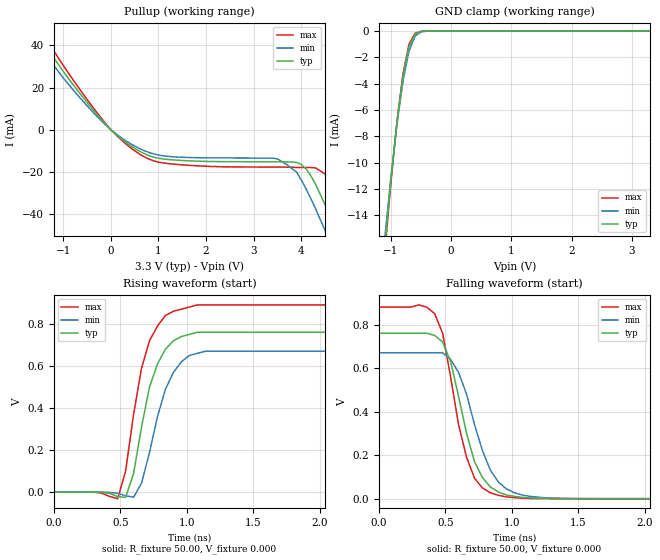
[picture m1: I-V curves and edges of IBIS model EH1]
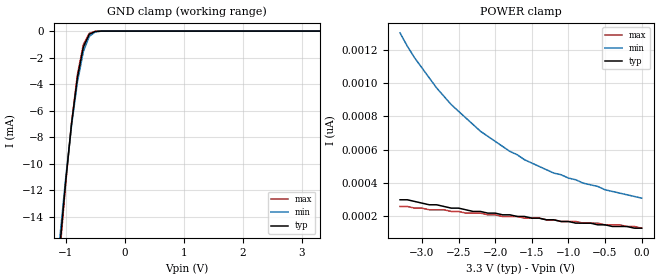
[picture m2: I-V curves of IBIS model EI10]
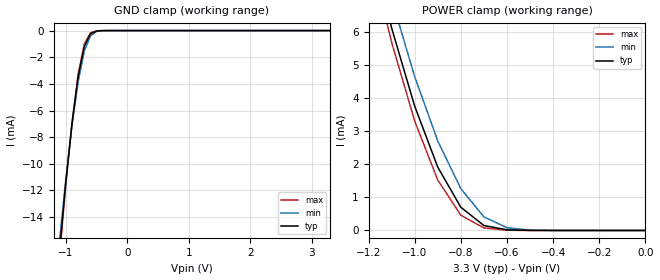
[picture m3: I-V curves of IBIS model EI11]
|   * fg1904b1.ibs * IBIS 2.1 Model file
| Rev History
| Rev No.   Description
| 1.0   3/22/07   Initial release with Updated Parasitic Parameters
|   Derived from fg1904ak ibis file
[IBIS Ver]   2.1
[Comment char]  |_char
[File name]   fg1904b1.ibs
[Date]   March 22, 2007
[File Rev]   1.0
[Source]   Originated at Integrated Device Technology, Inc.
[Disclaimer] (C) Copyright Integrated Device Technology, Inc. 2007
   All rights reserved
 hereby grants the user of this IBIS model a non-exclusive,
nontransferable license to use this IBIS model under the following terms.
Before using this IBIS model, the user should read this license.
If the user does not accept these terms,  the IBIS model should be
returned to IDT within 30 days.
   The user is granted this license only to use the IBIS model and
is not granted rights to sell, load, rent, lease or license the IBIS
model in whole or in part, or in modified form to anyone other than
user. User may modify the IBIS model to suit its specific
applications but rights to derivative works and such modifications
shall belong to IDT.
   This IBIS model is provided on an "AS IS" basis and IDT makes
absolutely no warranty with respect to the information contained
herein. IDT DISCLAIMS AND CUSTOMER WAIVES ALL WARRANTIES, EXPRESS
OR IMPLIED, INCLUDING WARRANTIES OF MERCHANTABILITY OR FITNESS FOR
A PARTICULAR PURPOSE. The entire risk as to quality and performance
is with the Customer. ACCORDINGLY, IN NO EVENT SHALL THE COMPANY BE
LIABLE FOR ANY DAMAGES, WHETHER IN CONTRACT OR TORT,INCLUDING ANY
LOST PROFITS OR OTHER INCIDENTAL, CONSEQUENTIAL, EXEMPLARY, OR
PUNITIVE DAMAGES ARISING OUT OF THE USE OR APPLICATION OF THE IBIS
model provided in this package. Further, IDT reserves the right to
make changes without notice to any product herein to improve
reliability, function, or design. IDT does not convey any license
under patent rights or any other intellectual property rights,
including those of third parties.
   IDT is not obligated to provide maintenance or support
for the licensed IBIS model.
|   COMPONENT: ICS9FG1904
[Component]   ICS9FG1904
[Manufacturer]  ICS
[Package]
| 72 lead QFN package
| variable   typ   min   max
R_pkg   332.1m   284.1m   380.1m
L_pkg   3.8165nH   2.9953nH   4.6377nH
C_pkg   0.3092pF   0.2316pF   0.3867pF
[Pin]   signal_name   model_name   R_pin   L_pin   C_pin
1   IREF   NC   0.3801  4.6377nH   0.3867pF
2   GNDA   GND   0.3681  4.4324nH   0.3673pF
3   VDDA   POWER   0.3561  4.2271nH   0.3479pF
4   HIGH_BW#   EI10   0.3441  4.0218nH   0.3285pF
5   FS_A_410   EI12   0.3321  3.8165nH   0.3092pF
6   DIF_0   EH1   0.3201  3.6112nH   0.2898pF
7   DIF_0#   EH1   0.3081  3.4059nH   0.2704pF
8   DIF_1   EH1   0.2961  3.2006nH   0.2510pF
9   DIF_1#   EH1   0.2841  2.9953nH   0.2316pF
10   GND   GND   0.2841  2.9953nH   0.2316pF
11   VDD   POWER   0.2961  3.2006nH   0.2510pF
12   DIF_2   EH1   0.3081  3.4059nH   0.2704pF
13   DIF_2#   EH1   0.3201  3.6112nH   0.2898pF
14   DIF_3   EH1   0.3321  3.8165nH   0.3092pF
15   DIF_3#   EH1   0.3441  4.0218nH   0.3285pF
16   DIF_4   EH1   0.3561  4.2271nH   0.3479pF
17   DIF_4#   EH1   0.3681  4.4324nH   0.3673pF
18   OE_01234#   EI8   0.3801  4.6377nH   0.3867pF
19   SMBCLK   EI8   0.3801  4.6377nH   0.3867pF
20   SMBDAT   EIOD1   0.3681  4.4324nH   0.3673pF
21   OE5#   EI8   0.3561  4.2271nH   0.3479pF
22   DIF_5   EH1   0.3441  4.0218nH   0.3285pF
23   DIF_5#   EH1   0.3321  3.8165nH   0.3092pF
24   OE6#   EI8   0.3201  3.6112nH   0.2898pF
25   DIF_6   EH1   0.3081  3.4059nH   0.2704pF
26   DIF_6#   EH1   0.2961  3.2006nH   0.2510pF
27   VDD   POWER   0.2841  2.9953nH   0.2316pF
28   GND   GND   0.2841  2.9953nH   0.2316pF
29   OE7#   EI8   0.2961  3.2006nH   0.2510pF
30   DIF_7   EH1   0.3081  3.4059nH   0.2704pF
31   DIF_7#   EH1   0.3201  3.6112nH   0.2898pF
32   OE8#   EI8   0.3321  3.8165nH   0.3092pF
33   DIF_8   EH1   0.3441  4.0218nH   0.3285pF
34   DIF_8#   EH1   0.3561  4.2271nH   0.3479pF
35   SMB_A0   EI10   0.3681  4.4324nH   0.3673pF
36   SMB_A1   EI10   0.3801  4.6377nH   0.3867pF
37   OE9#   EI8   0.3801  4.6377nH   0.3867pF
38   DIF_9   EH1   0.3681  4.4324nH   0.3673pF
39   DIF_9#   EH1   0.3561  4.2271nH   0.3479pF
40   OE10#   EI8   0.3441  4.0218nH   0.3285pF
41   DIF_10   EH1   0.3321  3.8165nH   0.3092pF
42   DIF_10#   EH1   0.3201  3.6112nH   0.2898pF
43   OE11#   EI8   0.3081  3.4059nH   0.2704pF
44   DIF_11   EH1   0.2961  3.2006nH   0.2510pF
45   DIF_11#   EH1   0.2841  2.9953nH   0.2316pF
46   GND   GND   0.2841  2.9953nH   0.2316pF
47   VDD   POWER   0.2961  3.2006nH   0.2510pF
48   OE12#   EI8   0.3081  3.4059nH   0.2704pF
49   DIF_12   EH1   0.3201  3.6112nH   0.2898pF
50   DIF_12#   EH1   0.3321  3.8165nH   0.3092pF
51   OE13#   EI8   0.3441  4.0218nH   0.3285pF
52   DIF_13   EH1   0.3561  4.2271nH   0.3479pF
53   DIF_13#   EH1   0.3681  4.4324nH   0.3673pF
54   OE14#   EI8   0.3801  4.6377nH   0.3867pF
55   DIF_14   EH1   0.3801  4.6377nH   0.3867pF
56   DIF_14#   EH1   0.3681  4.4324nH   0.3673pF
57   CKPWRGD/PD#   EI8   0.3561  4.2271nH   0.3479pF
58   DIF_15   EH1   0.3441  4.0218nH   0.3285pF
59   DIF_15#   EH1   0.3321  3.8165nH   0.3092pF
60   OE15_16#   EI8   0.3201  3.6112nH   0.2898pF
61   DIF_16   EH1   0.3081  3.4059nH   0.2704pF
62   DIF_16#   EH1   0.2961  3.2006nH   0.2510pF
63   VDD   POWER   0.2841  2.9953nH   0.2316pF
64   GND   GND   0.2841  2.9953nH   0.2316pF
65   DIF_17   EH1   0.2961  3.2006nH   0.2510pF
66   DIF_17#   EH1   0.3081  3.4059nH   0.2704pF
67   DIF_18   EH1   0.3201  3.6112nH   0.2898pF
68   DIF_18#   EH1   0.3321  3.8165nH   0.3092pF
69   OE17_18#   EI8   0.3441  4.0218nH   0.3285pF
70   CLK_IN   EI11   0.3561  4.2271nH   0.3479pF
71   CLK_IN#   EI11   0.3681  4.4324nH   0.3673pF
72   SMB_A2_PLLBYP#  EI10   0.3801  4.6377nH   0.3867pF
|** All model are simulated with typical corner process
[Diff Pin]   inv_pin   vdiff   tdelay_typ
6   7   NA   NA
8   9   NA   NA
12   13   NA   NA
14   15   NA   NA
16   17   NA   NA
22   23   NA   NA
25   26   NA   NA
30   31   NA   NA
33   34   NA   NA
38   39   NA   NA
41   42   NA   NA
44   45   NA   NA
49   50   NA   NA
52   53   NA   NA
55   56   NA   NA
58   59   NA   NA
61   62   NA   NA
65   66   NA   NA
67   68   NA   NA
70   71   NA   NA
| Models and submodels in the file (6): EH1 (Open_source), EI10 (Input), EI11 (Input), EI12 (Input), EI8 (Input), EIOD1 (I/O_open_drain)
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|   Model EH1
[Model]   EH1
Model_type   Open_source
Polarity   Inverting
C_comp   3.40pF   2.85pF   3.95pF
[Temperature Range]   27.00   70.00   0.000
[Voltage Range]   3.30V   3.00V   3.70V
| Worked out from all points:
|   slope of the pullup table from 0 to 0.495 V, typ, clamps not added: 56.2 ohm
|   GND clamp passes 1 mA (typ) near -0.68 V on its own axis
|   rising waveform, R_fixture 50.00, V_fixture 0.000: 20-80 % time 162ps typ, 177ps min, 159ps max; typ from 0 V to 0.76 V
|   falling waveform, R_fixture 50.00, V_fixture 0.000: 20-80 % time 187ps typ, 211ps min, 172ps max; typ from 0.76 V to 0 V
[Pullup]
| voltage   I(typ)   I(min)   I(max)
-3.3V     120mA      110mA      120mA
-1.9V     57.97mA    52.49mA    62.98mA
-1.5V     43.73mA    39.31mA    47.78mA
-100mV    2.37mA     2.07mA     2.66mA
800mV     -12.28mA   -10.8mA    -13.94mA
3.5V      -15.25mA   -13.83mA   -17.75mA
3.9V      -15.52mA   -20.05mA   -17.92mA
4.3V      -25.83mA   -37.4mA    -18.11mA
4.5V      -35.53mA   -47.74mA   -20.97mA
4.7V      -46.5mA    -58.63mA   -28.65mA
5.1V      -70.24mA   -81.19mA   -50.61mA
6.6V      -160mA     -170mA     -150mA
[GND_clamp]
| voltage   I(typ)   I(min)   I(max)
-3.3V     -160mA     -150mA     -160mA
-1.1V     -16.38mA   -15.67mA   -16.85mA
-1V       -11.38mA   -11.14mA   -11.54mA
-900mV    -6.99mA    -7.13mA    -6.92mA
-800mV    -3.48mA    -3.84mA    -3.27mA
-700mV    -1.2mA     -1.54mA    -1.01mA
-600mV    -240uA     -400uA     -170uA
-500mV    -29.28uA   -66.42uA   -17.31uA
-400mV    -2.53uA    -8.31uA    -1.16uA
3.3V      160pA      130nA      110pA
[Ramp]
| variable   typ   min   max
dV/dt_r   0.46/0.16n   0.40/0.17n   0.53/0.15n
dV/dt_f   0.45/0.18n   0.40/0.21n   0.53/0.16n
R_load = 50.00
[Rising Waveform]
R_fixture = 50.00
V_fixture = 0.000
V_fixture_min = 0.000
V_fixture_max = 0.000
| time   V(typ)   V(min)   V(max)
0s        0V         0V         0V
480ps     -20.67mV   -5.16mV    -30.74mV
540ps     -24.54mV   -16.6mV    100mV
600ps     89.11mV    -23.72mV   370mV
660ps     310mV      43mV       590mV
720ps     500mV      190mV      720mV
840ps     680mV      490mV      840mV
900ps     720mV      570mV      860mV
1.14ns    760mV      670mV      890mV
3ns       760mV      670mV      890mV
[Falling Waveform]
R_fixture = 50.00
V_fixture = 0.000
V_fixture_min = 0.000
V_fixture_max = 0.000
| time   V(typ)   V(min)   V(max)
0s        760mV      670mV      880mV
420ps     750mV      670mV      850mV
480ps     720mV      670mV      760mV
540ps     630mV      640mV      560mV
660ps     300mV      480mV      190mV
720ps     170mV      340mV      93.8mV
840ps     53.28mV    130mV      26.91mV
960ps     17.18mV    44.94mV    8.25mV
1.14ns    3.66mV     10.53mV    1.07mV
3ns       3.63uV     6.1uV      2.47uV
|   Model EI10
[Model]   EI10
Model_type   Input
Polarity   Non-Inverting
Enable   Active-High
Vinl =   0.80V
Vinh =   2.00V
C_comp   3.40pF   2.85pF   3.95pF
[Temperature Range]   27.00   70.00   0.000
[Voltage Range]   3.30V   3.00V   3.70V
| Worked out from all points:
|   GND clamp passes 1 mA (typ) near -0.68 V on its own axis
[GND_clamp]
| voltage   I(typ)   I(min)   I(max)
-3.3V     -160mA     -150mA     -160mA
-1.1V     -16.38mA   -15.67mA   -16.85mA
-1V       -11.38mA   -11.14mA   -11.54mA
-900mV    -6.99mA    -7.13mA    -6.92mA
-800mV    -3.48mA    -3.84mA    -3.27mA
-700mV    -1.2mA     -1.54mA    -1.01mA
-600mV    -240uA     -400uA     -170uA
-500mV    -29.28uA   -66.42uA   -17.31uA
-400mV    -2.53uA    -8.31uA    -1.16uA
3.3V      160pA      130nA      110pA
[POWER_clamp]
| voltage   I(typ)   I(min)   I(max)
-3.3V     300pA      1.3nA      260pA
-3.1V     290pA      1.15nA     250pA
-2.9V     270pA      1.03nA     240pA
-2.8V     270pA      970pA      240pA
-2.6V     250pA      870pA      230pA
-2.2V     230pA      710pA      220pA
-1.8V     210pA      590pA      200pA
-1.2V     180pA      460pA      180pA
-900mV    160pA      420pA      170pA
-500mV    150pA      360pA      150pA
-300mV    140pA      340pA      150pA
0V        130pA      310pA      130pA
|   Model EI11
[Model]   EI11
Model_type   Input
Polarity   Non-Inverting
Vinl =   0.80V
Vinh =   2.00V
C_comp   3.40pF   2.85pF   3.95pF
[Temperature Range]   27.00   70.00   0.000
[Voltage Range]   3.30V   3.00V   3.70V
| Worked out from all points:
|   GND clamp passes 1 mA (typ) near -0.68 V on its own axis
|   POWER clamp passes 1 mA (typ) near -0.82 V on its own axis
[GND_clamp]
| voltage   I(typ)   I(min)   I(max)
-3.3V     -160mA     -150mA     -160mA
-1.1V     -16.38mA   -15.67mA   -16.85mA
-1V       -11.38mA   -11.14mA   -11.54mA
-900mV    -6.99mA    -7.13mA    -6.92mA
-800mV    -3.48mA    -3.84mA    -3.27mA
-700mV    -1.2mA     -1.54mA    -1.01mA
-600mV    -240uA     -400uA     -170uA
-500mV    -29.28uA   -66.42uA   -17.31uA
-400mV    -2.53uA    -8.31uA    -1.16uA
3.3V      160pA      130nA      110pA
[POWER_clamp]
| voltage   I(typ)   I(min)   I(max)
-3.3V     130mA      120mA      140mA
-1.2V     8.92mA     9.69mA     8.55mA
-1.1V     6.11mA     6.99mA     5.68mA
-1V       3.75mA     4.64mA     3.3mA
-900mV    1.91mA     2.7mA      1.52mA
-800mV    700uA      1.26mA     460uA
-700mV    150uA      410uA      77.11uA
-600mV    19.94uA    82.32uA    8.03uA
-500mV    1.95uA     11.93uA    590nA
0V        160pA      550pA      150pA
